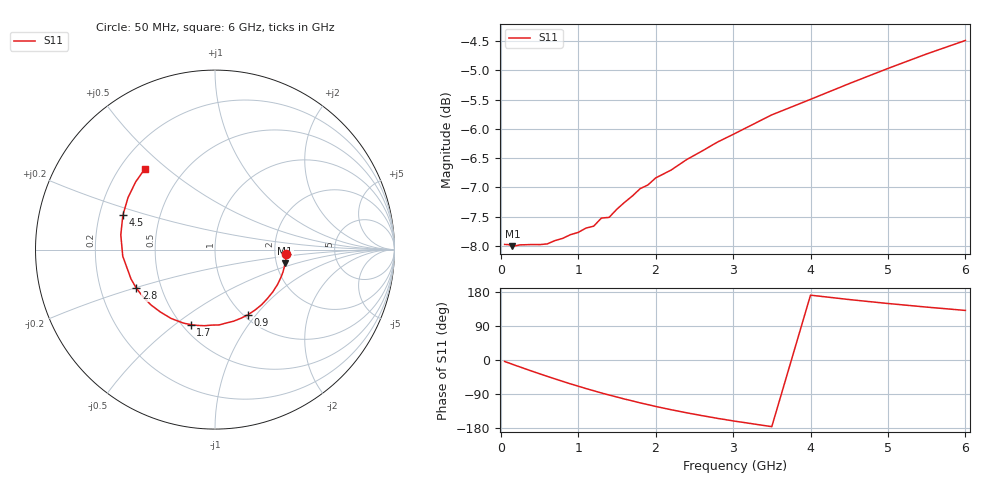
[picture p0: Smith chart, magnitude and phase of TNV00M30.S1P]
! SIEMENS Discrete & RF Semiconductors
! BAS70-07W
! Si Schottky Diode in SOT343
! IF = 0.3 mA
! S-Parameters:  February  1997
# GHz  S  MA  R  50
!  f  S11
! GHz  MAG  ANG
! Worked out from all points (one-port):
!   34 points, 50 MHz to 6 GHz, reference 50 ohm
!   lowest |S11| = -8.0 dB at 150 MHz (marker M1), VSWR 2.32, Z = 111 - j20.4 ohm
!   |S11| at or under -10 dB: nowhere
!   S11 on the Smith chart (normalised r, x): 50 MHz: 2.32, -0.15; 900 MHz: 1.05, -0.91; 1.7 GHz: 0.55, -0.57; 2.8 GHz: 0.36, -0.20; 4.5 GHz: 0.30, +0.16; 6 GHz: 0.30, +0.42
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0.05  0.3991 -3.9
0.15  0.3977 -11.2
0.25  0.3988 -18.4
0.4  0.399 -29.2
0.6  0.3995 -43.1
0.7  0.4021 -49.8
0.8  0.4039 -56.4
0.9  0.4068 -63.0
1.1  0.4122 -75.3
1.2  0.4137 -81.1
1.3  0.4204 -87.0
1.4  0.421 -92.4
1.5  0.4279 -97.7
1.6  0.4337 -103.1
1.7  0.4391 -107.9
1.8  0.4455 -113.2
2  0.455 -122.6
2.2  0.4621 -131.2
2.4  0.4717 -139.3
2.6  0.4798 -146.8
2.8  0.4884 -154.0
3  0.4957 -160.7
3.5  0.5153 -175.9
4  0.5312 171.1
4.5  0.548 159.5
5  0.5646 149.1
5.5  0.581 139.6
6  0.5966 130.8
